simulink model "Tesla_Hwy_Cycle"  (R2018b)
settings: Solver=VariableStepAuto  StartTime=0.0  StopTime=765  FixedStep=1e-3  RelTol=1e-3
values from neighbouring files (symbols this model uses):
  B = 0    [Tesla_Initialization.m]    (also in PMSM_EV_init_v2.m; Leaf_Initialization.m)
  J = 0.3    [Tesla_Initialization.m]    (also in PMSM_EV_init_v2.m; Leaf_Initialization.m)
  P = 8    [Tesla_Initialization.m]    (also in PMSM_EV_init_v2.m; Iqbal Husain - Example12_1.m = V.*I; Leaf_Initialization.m)
  Rs = 0.046    [Tesla_Initialization.m]    (also in PMSM_EV_init_v2.m; Leaf_Initialization.m)
  Speed = [+0.000000E+00	+6.054730E+02	+1.210946E+03	+1.816419E+03	+2.421892E+03	+3.027365E+03	+3.632838E+03	+4.238311E+03	+5.775695E+03	+7.313079E+03	+8.850463E+03	+1.038785E+04	+1.192523E+04	+1.346262E+04	+1.500000E+04]    [PMSM_EV_init_v2.m]
  Tesla_id_axis = [-8.764242E+02	-7.790438E+02	-6.816633E+02	-5.842828E+02	-4.869024E+02	-3.895219E+02	-2.921414E+02	-1.947609E+02	-9.738047E+01	+0.000000E+00]    [Tesla_Initialization.m]
  Tesla_iq_axis = [+0.000000E+00	+9.738047E+01	+1.947609E+02	+2.921414E+02	+3.895219E+02	+4.869024E+02	+5.842828E+02	+6.816633E+02	+7.790438E+02	+8.764242E+02]    [Tesla_Initialization.m]
  Tesla_Ld = [+8.821895E-05	+8.924938E-05	+9.139742E-05	+9.462732E-05	+1.042993E-04	+1.207302E-04	+1.435858E-04	+1.651379E-04	+1.771179E-04	+1.815302E-04    [Tesla_Initialization.m]
  Tesla_Lq = [+2.750008E-04	+2.848007E-04	+2.919706E-04	+2.981362E-04	+3.048757E-04	+3.200995E-04	+3.552424E-04	+3.955550E-04	+4.296280E-04	+4.500669E-04    [Tesla_Initialization.m]
  Tesla_omega_axis = [+0.000000E+00	+6.292573E+01	+1.258515E+02	+1.887772E+02	+2.517029E+02	+3.146286E+02	+3.775544E+02	+4.404801E+02	+5.271540E+02	+6.138279E+02	+7.005019E+02	+7.871758E+02	+8.738497E+02	+9.605236E+02	+1.047198E+03]    [Tesla_Initialization.m]
  Tesla_phid = [-9.964313E-02	-8.749389E-02	-7.506085E-02	-6.231998E-02	-4.899731E-02	-3.359246E-02	-1.574417E-02	+5.955898E-03	+2.974036E-02	+5.474011E-02    [Tesla_Initialization.m]
  Tesla_phiq = [+1.577834E-05	+2.291095E-05	+1.626960E-05	+6.018524E-06	+7.523247E-06	+1.073346E-05	+2.148179E-05	+1.486713E-05	+9.491501E-06	-7.613491E-07    [Tesla_Initialization.m]
  Tesla_T = [+1.173389E-01	+1.514507E-01	+9.410508E-02	+2.983867E-02	+3.108232E-02	+3.547627E-02	+5.325126E-02	+2.456943E-02	+7.842834E-03	+0.000000E+00    [Tesla_Initialization.m]
  Tesla_torque_axis = [+0.000000E+00	+2.093141E+01	+4.186282E+01	+6.279422E+01	+8.372563E+01	+1.046570E+02	+1.255884E+02	+1.396842E+02	+1.571452E+02	+1.795502E+02	+2.098144E+02	+2.538064E+02	+3.242133E+02	+4.360097E+02]    [Tesla_Initialization.m]
  Torque = [+0.000000E+00	+7.333624E+00	+1.466725E+01	+2.200087E+01	+2.933450E+01	+3.666812E+01	+4.400174E+01	+5.043561E+01	+5.870849E+01	+6.980054E+01	+8.566293E+01	+1.107686E+02	+1.535327E+02	+2.089386E+02]    [PMSM_EV_init_v2.m]
undefined symbols (not defined in the file or in its folder): A1, B766, HEV_Param
libraries: fl_lib x18, nesl_utility x9, sdl_lib x4

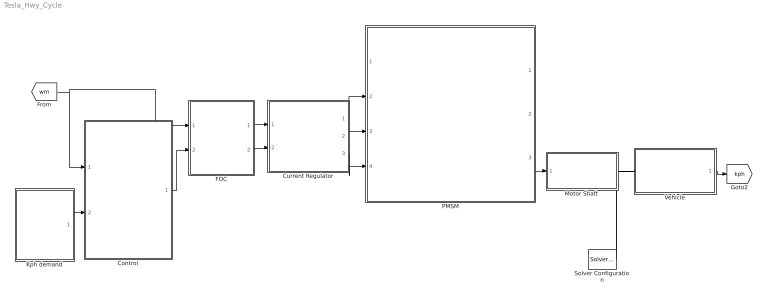
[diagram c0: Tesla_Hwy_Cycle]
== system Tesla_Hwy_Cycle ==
  Control : Subsystem
  Current Regulator : Subsystem
  FOC : Subsystem
  Kph demand : Subsystem
  Motor Shaft : Subsystem
  PMSM : Subsystem
  Solver Configuration : nesl_utility/Solver Configuration  PhysicalDomain=network_engine_domain  SubClassName=solver  LeftPortType=input  RightPortType=generic  Tones=[]  Harmonics=[]  SimulateNoise=off  Profile=off  UseLocalSampling=off  EnableSwitchedLinearOptims=on  FrequencyDomain=off  UseCCode=off  RelTol=0.001  AbsTol=1e-06  MinStep=1e-09  ToWorkspace=off  RevertToSquareIcSolve=off  NumHomotopyIterations=100  PhasorMode=off  PhasorModeNumHarmonics=1  DoDC=off  ResidualTolerance=1e-09  UseLocalSolver=off  LocalSolverChoice=NE_BACKWARD_EULER_ADVANCER  LocalSolverSampleTime=0.001  DoFixedCost=off  MaxNonlinIter=3  MaxModeIter=2  LinearAlgebra=auto  EquationFormulation=NE_TIME_EF  DelaysMemoryBudget=1024  AutomaticFiltering=on  FilteringTimeConstant=0.001  PartitionStorageMethod=AS_NEEDED  PartitionMemoryBudget=1024
  Vehicle : Subsystem
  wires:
  [wm] -> FOC/1(Speed), Control/1("rad/s ")
  FOC/2(Id_ref) -> Current Regulator/2(id_ref)
  PMSM/3(Torque (Nm)) -> Motor Shaft/1(In1)
  Current Regulator/2(Vb) -> PMSM/3(Vb)
  Control/1(Mot_TReq) -> FOC/2(Torque)
  Current Regulator/3(Vc) -> PMSM/4(Vc)
  Kph demand/1(Acc) -> Control/2(Acc)
  FOC/1(Iq_ref) -> Current Regulator/1(iq_ref)
  Vehicle/1(VehSpd) -> [kph]
  Current Regulator/1(Va) -> PMSM/2(Va)
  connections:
  Vehicle/LConn1 -- Solver Configuration/RConn1 -- Motor Shaft/RConn1

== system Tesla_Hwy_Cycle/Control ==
  "rad/s " : Inport
  Acc : Inport  Port=2
  Convert acceleration demand to motor speed demand. : Lookup  InputValues=[0 30]  Table=[0 10000]
  Gain : Gain  Gain=60/(2*pi)
  Motor Controller : Subsystem
  Mot_TReq : Outport
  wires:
  Motor Controller/1(M_Trq_Dem) -> Mot_TReq/1
  Convert acceleration demand to motor speed demand./1 -> Motor Controller/1(Mot_RPM_Dem)
  "rad/s "/1 -> Gain/1
  Acc/1 -> Convert acceleration demand to motor speed demand./1
  Gain/1 -> Motor Controller/2(Mot_RPM)

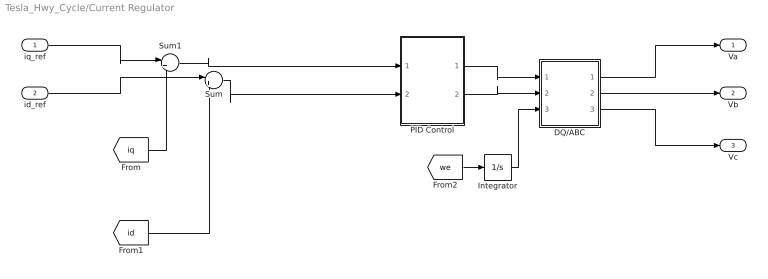
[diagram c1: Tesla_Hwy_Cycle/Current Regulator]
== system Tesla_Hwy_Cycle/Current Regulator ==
  iq_ref : Inport
  id_ref : Inport  Port=2
  DQ/ABC : Subsystem
  Integrator : Integrator
  PID Control : Subsystem
  Sum : Sum  Inputs=|+-
  Sum1 : Sum  Inputs=|+-
  Va : Outport
  Vb : Outport  Port=2
  Vc : Outport  Port=3
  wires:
  [iq] -> Sum1/2
  [id] -> Sum/2
  PID Control/1(Out1) -> DQ/ABC/1(Vq)
  Sum/1 -> PID Control/2(In3)
  PID Control/2(Out2) -> DQ/ABC/2(Vd)
  id_ref/1 -> Sum/1
  [we] -> Integrator/1
  iq_ref/1 -> Sum1/1
  Integrator/1 -> DQ/ABC/3(theta_rf)
  Sum1/1 -> PID Control/1(In1)
  DQ/ABC/1(Va) -> Va/1
  DQ/ABC/2("Vb ") -> Vb/1
  DQ/ABC/3("Vc ") -> Vc/1

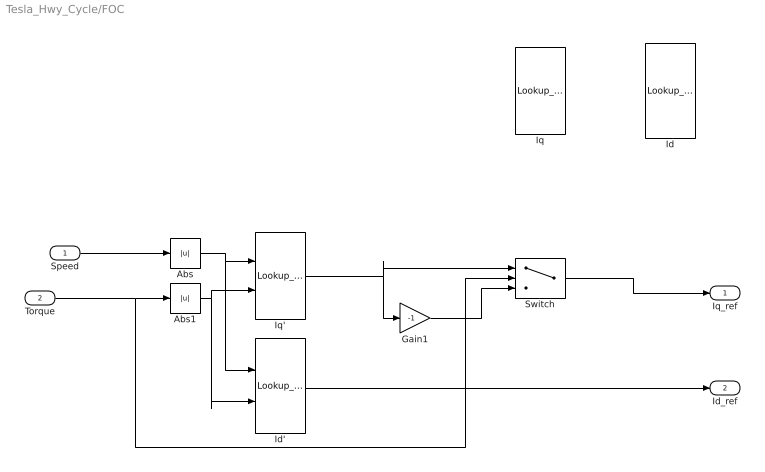
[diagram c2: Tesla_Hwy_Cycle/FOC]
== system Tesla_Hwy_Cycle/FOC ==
  Speed : Inport
  Torque : Inport  Port=2
  Abs : Abs
  Abs1 : Abs
  Gain1 : Gain  Gain=-1
  Id : Lookup_n-D  Commented=on  BreakpointsForDimension1=Speed  BreakpointsForDimension2=Torque  Table=Id_C'  InternalRulePriority=Speed  RndMeth=Simplest
  Id' : Lookup_n-D  BreakpointsForDimension1=Tesla_omega_axis  BreakpointsForDimension2=Tesla_torque_axis  Table=Tesla_Id'  InternalRulePriority=Speed  RndMeth=Simplest
  Iq : Lookup_n-D  Commented=on  BreakpointsForDimension1=Speed  BreakpointsForDimension2=Torque  Table=Iq_C'  InternalRulePriority=Speed  RndMeth=Simplest
  Iq' : Lookup_n-D  BreakpointsForDimension1=Tesla_omega_axis  BreakpointsForDimension2=Tesla_torque_axis  Table=Tesla_Iq'  InternalRulePriority=Speed  RndMeth=Simplest
  Switch : Switch  Criteria=u2 > Threshold
  Iq_ref : Outport
  Id_ref : Outport  Port=2
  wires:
  Abs/1 -> Id'/1, Iq'/1
  Abs1/1 -> Id'/2, Iq'/2
  Speed/1 -> Abs/1
  Switch/1 -> Iq_ref/1
  Torque/1 -> Switch/2, Abs1/1
  Gain1/1 -> Switch/3
  Iq'/1 -> Switch/1, Gain1/1
  Id'/1 -> Id_ref/1

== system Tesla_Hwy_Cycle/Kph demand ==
  From Spreadsheet3 : FromSpreadsheet  FileName=Highway_cycle.xlsx  Range=A1:B766  ExtrapolationBeforeFirstDataPoint=Hold first value
  Gain : Gain  Gain=1.6
  Vehicle Speed Controller : Subsystem
  Acc : Outport
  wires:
  From Spreadsheet3/1 -> Gain/1
  [kph] -> Vehicle Speed Controller/2(Veh Spd)
  Gain/1 -> Vehicle Speed Controller/1(Ref Spd)
  Vehicle Speed Controller/1(Acc) -> Acc/1

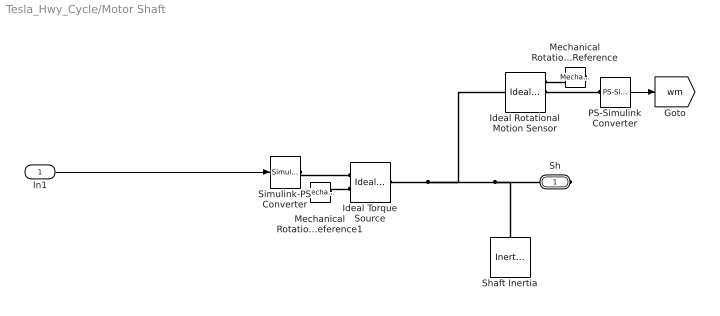
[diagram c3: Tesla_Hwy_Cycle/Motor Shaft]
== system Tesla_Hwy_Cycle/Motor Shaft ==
  In1 : Inport
  Ideal Rotational Motion Sensor : fl_lib/Mechanical/Mechanical Sensors/Ideal Rotational Motion Sensor  offset=0 rad
  Ideal Torque Source : fl_lib/Mechanical/Mechanical Sources/Ideal Torque Source
  Mechanical Rotational Reference : fl_lib/Mechanical/Rotational Elements/Mechanical Rotational Reference
  Mechanical Rotational Reference1 : fl_lib/Mechanical/Rotational Elements/Mechanical Rotational Reference
  PS-Simulink Converter : nesl_utility/PS-Simulink Converter  PhysicalDomain=network_engine_domain  SubClassName=ps_output  LeftPortType=input  RightPortType=output  PseudoPeriodic=off  Frequencies=[]  Unit=rad/s  AffineConversion=off
  Shaft Inertia : fl_lib/Mechanical/Rotational Elements/Inertia  inertia=HEV_Param.Motor.Shaft_Inertia kg*m^2  w_specify=on  w_priority=High  w=0 rad/s  w_nominal_specify=off  w_nominal_unit=rad/s  w_nominal_value=1  t_specify=off  t_priority=High  t=0 N*m  t_nominal_specify=off  t_nominal_unit=N*m  t_nominal_value=1
  Simulink-PS Converter : nesl_utility/Simulink-PS Converter  PhysicalDomain=network_engine_domain  SubClassName=ps_input  LeftPortType=input  RightPortType=output  PseudoPeriodic=off  Frequencies=[]  NoiseDistribution=none  NoiseParameters=[]  Unit=1  AffineConversion=off  FilteringAndDerivatives=zero  SimscapeFilterOrder=1  InputFilterTimeConstant=.001  UdotUserProvided=0
  Sh : PMIOPort  Side=Right
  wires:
  In1/1 -> Simulink-PS Converter/1
  PS-Simulink Converter/1 -> [wm]
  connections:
  Mechanical Rotational Reference1/LConn1 -- Ideal Torque Source/RConn2
  Ideal Torque Source/LConn1 -- Ideal Rotational Motion Sensor/LConn1 -- Shaft Inertia/LConn1 -- Sh/RConn1
  Simulink-PS Converter/RConn1 -- Ideal Torque Source/RConn1
  Mechanical Rotational Reference/LConn1 -- Ideal Rotational Motion Sensor/RConn1
  PS-Simulink Converter/LConn1 -- Ideal Rotational Motion Sensor/RConn2

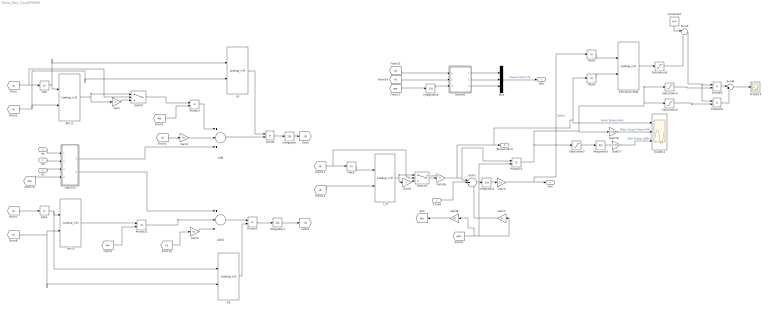
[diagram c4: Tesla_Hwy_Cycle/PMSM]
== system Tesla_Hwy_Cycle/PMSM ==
  T_load : Inport
  Va : Inport  Port=2
  Vb : Inport  Port=3
  Vc : Inport  Port=4
  ABC/DQ : Subsystem
  Abs{,1..2,5..6} (5 alike) : Abs
  Add : Sum  Inputs=+-+
  Add1 : Sum  Inputs=+--
  Constant2 : Constant  Value=1e-6
  DQ/ABC : Subsystem
  Divide : Product  Inputs=/*
  Divide1 : Product  Inputs=*/
  Divide4 : Product  Inputs=/*
  Efficiency Map : Lookup_n-D  BreakpointsForDimension1=Tesla_omega_axis  BreakpointsForDimension2=Tesla_torque_axis  Table=Tesla_eff'  ExtrapMethod=Clip  UseLastTableValue=on  InternalRulePriority=Speed  RndMeth=Simplest
  Gain : Gain  Gain=-1
  Gain1 : Gain  Gain=Rs
  Gain16 : Gain
  Gain17 : Gain  Gain=2.77778e-7
  Gain18 : Gain  Gain=1/1000
  Gain2 : Gain  Gain=Rs
  Gain3 : Gain  Gain=-1
  Gain4 : Gain  Gain=1/J
  Gain7 : Gain  Gain=B
  Gain8 : Gain  Gain=P/2
  Integrator{,1..2,4..5} (5 alike) : Integrator
  Ld : Lookup_n-D  BreakpointsForDimension1=Tesla_iq_axis  BreakpointsForDimension2=Tesla_id_axis  Table=Tesla_Ld  InternalRulePriority=Speed  RndMeth=Simplest
  Lq : Lookup_n-D  BreakpointsForDimension1=Tesla_iq_axis  BreakpointsForDimension2=Tesla_id_axis  Table=Tesla_Lq  InternalRulePriority=Speed  RndMeth=Simplest
  Mux : Mux  Inputs=3
  Product{,1,3,9} (4 alike) : Product
  Saturation2 : Saturate  UpperLimit=inf  LowerLimit=0
  Saturation3 : Saturate  UpperLimit=inf  LowerLimit=0
  Saturation4 : Saturate  UpperLimit=0  LowerLimit=-inf
  Saturation5 : Saturate  UpperLimit=inf  LowerLimit=0.1
  Scope12 : Scope  NumInputPorts=3
  Scope13 : Scope
  Sum1 : Sum  Inputs=|+--
  Sum5 : Sum  Inputs=|++
  Sum6 : Sum  Inputs=|++
  Switch : Switch  Criteria=u2 > Threshold
  Switch1 : Switch  Criteria=u2 > Threshold
  T_m : Lookup_n-D  BreakpointsForDimension1=Tesla_iq_axis  BreakpointsForDimension2=Tesla_id_axis  Table=Tesla_T  ExtrapMethod=Clip  UseLastTableValue=on  InternalRulePriority=Speed  RndMeth=Simplest
  phi_d : Lookup_n-D  BreakpointsForDimension1=Tesla_iq_axis  BreakpointsForDimension2=Tesla_id_axis  Table=Tesla_phid  InternalRulePriority=Speed  RndMeth=Simplest
  phi_q : Lookup_n-D  BreakpointsForDimension1=Tesla_iq_axis  BreakpointsForDimension2=Tesla_id_axis  Table=Tesla_phiq  InternalRulePriority=Speed  RndMeth=Simplest
  iabc : Outport
  wm : Outport  Port=2
  Torque (Nm) : Outport  Port=3
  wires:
  phi_d/1 -> Product1/1
  [iq] -> Abs1/1
  Divide1/1 -> Integrator1/1
  [we] -> ABC/DQ/4(omega_rf)
  T_m/1 -> Gain3/1, Switch1/1
  [id] -> Lq/2, phi_d/2
  [id] -> Ld/2, phi_q/2
  Vb/1 -> ABC/DQ/2(Vb)
  Integrator4/1 -> DQ/ABC/3(theta_rf)
  [id] -> Gain1/1
  Product1/1 -> Add1/2
  [we] -> Integrator4/1
  [iq] -> DQ/ABC/1(Iq)
  Abs/1 -> Ld/1, phi_q/1
  Vc/1 -> ABC/DQ/3(Vc)
  Gain4/1 -> Abs5/1, wm/1  "Speed"
  Divide/1 -> Integrator/1
  Add1/1 -> Divide1/1
  Gain1/1 -> Add/2
  [id] -> DQ/ABC/2(Id)
  Abs1/1 -> Lq/1, phi_d/1
  [iq] -> Gain2/1
  ABC/DQ/2("q ") -> Add1/1
  Integrator2/1 -> Gain4/1
  Ld/1 -> Divide/1
  [we] -> Product/2
  phi_q/1 -> Gain/1, Switch/1
  Product/1 -> Add/1
  Integrator1/1 -> [iq]
  ABC/DQ/1(d) -> Add/3
  T_load/1 -> Sum1/2
  [iq] -> Switch/2, Abs/1
  Add/1 -> Divide/2
  Switch1/1 -> Gain16/1  "Torque(Nm)"
  Switch/1 -> Product/1
  Sum1/1 -> Integrator2/1
  Abs2/1 -> T_m/1
  [we] -> Product1/2
  Va/1 -> ABC/DQ/1(Va)
  Integrator/1 -> [id]
  Gain/1 -> Switch/3
  Lq/1 -> Divide1/2
  Mux/1 -> iabc/1  "Phase Current (A)"
  Gain3/1 -> Switch1/3
  Gain2/1 -> Add1/3
  DQ/ABC/2("Ib ") -> Mux/2
  DQ/ABC/3("Ic ") -> Mux/3
  [wm] -> Gain7/1, Product3/2, Gain8/1
  Gain7/1 -> Sum1/3
  Gain8/1 -> [we]
  [id] -> T_m/2
  DQ/ABC/1(Ia) -> Mux/1
  [iq] -> Abs2/1, Switch1/2
  Gain16/1 -> Abs6/1, Scope12/1, Torque (Nm)/1, Product3/1, Sum1/1  "Motor Torque (Nm)"
  Integrator5/1 -> Gain17/1
  Gain18/1 -> Scope12/2  "Motor Output Power (kW)"
  Saturation2/1 -> Integrator5/1
  Gain17/1 -> Scope12/3  "Total Energy (kWhr)"
  Abs5/1 -> Efficiency Map/1
  Abs6/1 -> Efficiency Map/2
  Saturation4/1 -> Product9/2
  Saturation3/1 -> Divide4/2
  Product9/1 -> Sum6/2
  Sum6/1 -> Scope13/1
  Sum5/1 -> Product9/1, Divide4/1
  Constant2/1 -> Sum5/1
  Divide4/1 -> Sum6/1
  Product3/1 -> Saturation4/1, Saturation3/1, Gain18/1, Saturation2/1
  Efficiency Map/1 -> Saturation5/1
  Saturation5/1 -> Sum5/2

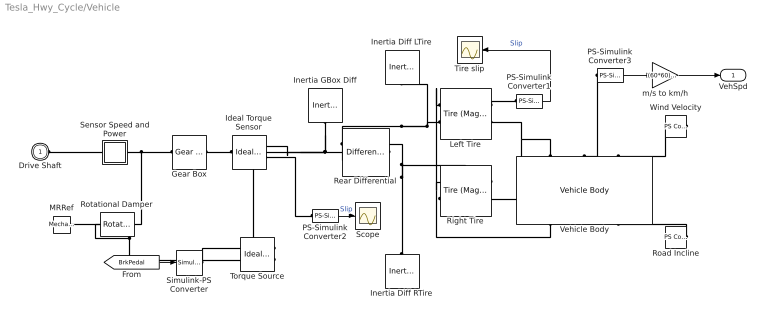
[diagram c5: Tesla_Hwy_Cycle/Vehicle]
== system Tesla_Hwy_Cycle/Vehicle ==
  Gear Box : fl_lib/Mechanical/Mechanisms/Gear Box  ratio=HEV_Param.Vehicle.Engine_Vehicle_Gear_Ratio  t_in_specify=off  t_in_priority=High  t_in=0 N*m  t_in_nominal_specify=off  t_in_nominal_unit=N*m  t_in_nominal_value=1  t_out_specify=off  t_out_priority=High  t_out=0 N*m  t_out_nominal_specify=off  t_out_nominal_unit=N*m  t_out_nominal_value=1
  Ideal Torque Sensor : fl_lib/Mechanical/Mechanical Sensors/Ideal Torque Sensor
  Inertia Diff LTire : fl_lib/Mechanical/Rotational Elements/Inertia  inertia=HEV_Param.Vehicle.Wheel_Inertia*2 kg*m^2  w_specify=on  w_priority=High  w=0 rad/s  w_nominal_specify=off  w_nominal_unit=rad/s  w_nominal_value=1  t_specify=off  t_priority=High  t=0 N*m  t_nominal_specify=off  t_nominal_unit=N*m  t_nominal_value=1
  Inertia Diff RTire : fl_lib/Mechanical/Rotational Elements/Inertia  inertia=HEV_Param.Vehicle.Wheel_Inertia*2 kg*m^2  w_specify=on  w_priority=High  w=0 rad/s  w_nominal_specify=off  w_nominal_unit=rad/s  w_nominal_value=1  t_specify=off  t_priority=High  t=0 N*m  t_nominal_specify=off  t_nominal_unit=N*m  t_nominal_value=1
  Inertia GBox Diff : fl_lib/Mechanical/Rotational Elements/Inertia  inertia=HEV_Param.Vehicle.Trans.Inertia kg*m^2  w_specify=on  w_priority=High  w=0 rad/s  w_nominal_specify=off  w_nominal_unit=rad/s  w_nominal_value=1  t_specify=off  t_priority=High  t=0 N*m  t_nominal_specify=off  t_nominal_unit=N*m  t_nominal_value=1
  Left Tire : sdl_lib/Tires & Vehicles/Tire (Magic Formula)  parameterization=1  F_z1=HEV_Param.Vehicle.Tire.Rated_Vertical_Load N  F_x1=HEV_Param.Vehicle.Tire.Rated_Peak_Long_Force N  kappa1=HEV_Param.Vehicle.Tire.Slip_At_Peak_Force  B_m=10  C_m=1.9  D_m=1  E_m=0.97  fz0=4e+3 N  p_Cx=1.685  p_Dx=[ 1.21 -0.037 ]  p_Ex=[ 0.344 0.095 -0.02 0 ]  p_Kx=[ 21.51 -0.163 0.245 ]  p_Hx=[ -0.002 0.002 ]  p_Vx=[ 0 0 ]  v_tr_thr=0.1 m/s  r_e=HEV_Param.Vehicle.Tire_Radius m  model_compliance=0  stiffness=1e+6 N/m  damping=1000 N/(m/s)  model_inertia=1  inertia=1e-2 kg*m^2  initial_velocity=0 rpm  model_resistance=1  resistance_model=1  coeff=0.015  p_tire=250e3 Pa  alpha=-0.003  beta=0.97  coeff_a=84e-4  coeff_b=6.2e-4 s/m  coeff_c=1.6e-4 s^2/m^2  v_thr=1e-3 m/s
  MRRef : fl_lib/Mechanical/Rotational Elements/Mechanical Rotational Reference
  PS-Simulink Converter1 : nesl_utility/PS-Simulink Converter  PhysicalDomain=network_engine_domain  SubClassName=ps_output  LeftPortType=input  RightPortType=output  PseudoPeriodic=off  Frequencies=[]  Unit=1  AffineConversion=off
  PS-Simulink Converter2 : nesl_utility/PS-Simulink Converter  PhysicalDomain=network_engine_domain  SubClassName=ps_output  LeftPortType=input  RightPortType=output  PseudoPeriodic=off  Frequencies=[]  Unit=1  AffineConversion=off
  PS-Simulink Converter3 : nesl_utility/PS-Simulink Converter  PhysicalDomain=network_engine_domain  SubClassName=ps_output  LeftPortType=input  RightPortType=output  PseudoPeriodic=off  Frequencies=[]  Unit=m/s  AffineConversion=off
  Rear Differential : sdl_lib/Gears/Differential  driveshaft_location=2  cd_ratio=1  friction_model=1  efficiency=[ 0.85 0.92 ]  mu_visc=[ 0 0 ] N*m/(rad/s)  pwr_thr=[ 0.001 0.001 ] W  carrier_inertia=0 kg*m^2  planet_inertia=0 kg*m^2  temperature_TLU=[ 280 300 320 ] K  efficiency_ss_TLU=[ 0.95 0.9 0.85 ]  efficiency_cd_TLU=[ 0.95 0.9 0.85 ]  thermal_mass=50 J/K  T_init=300 K
  Right Tire : sdl_lib/Tires & Vehicles/Tire (Magic Formula)  parameterization=1  F_z1=HEV_Param.Vehicle.Tire.Rated_Vertical_Load N  F_x1=HEV_Param.Vehicle.Tire.Rated_Peak_Long_Force N  kappa1=HEV_Param.Vehicle.Tire.Slip_At_Peak_Force  B_m=10  C_m=1.9  D_m=1  E_m=0.97  fz0=4e+3 N  p_Cx=1.685  p_Dx=[ 1.21 -0.037 ]  p_Ex=[ 0.344 0.095 -0.02 0 ]  p_Kx=[ 21.51 -0.163 0.245 ]  p_Hx=[ -0.002 0.002 ]  p_Vx=[ 0 0 ]  v_tr_thr=0.1 m/s  r_e=HEV_Param.Vehicle.Tire_Radius m  model_compliance=0  stiffness=1e+6 N/m  damping=1000 N/(m/s)  model_inertia=1  inertia=1e-2 kg*m^2  initial_velocity=0 rpm  model_resistance=1  resistance_model=1  coeff=0.015  p_tire=250e3 Pa  alpha=-0.003  beta=0.97  coeff_a=84e-4  coeff_b=6.2e-4 s/m  coeff_c=1.6e-4 s^2/m^2  v_thr=1e-3 m/s
  Road Incline : fl_lib/Physical Signals/Sources/PS Constant  constant=HEV_Param.Vehicle.Incline
  Rotational Damper : fl_lib/Mechanical/Rotational Elements/Rotational Damper  D=HEV_Param.Vehicle.Trans.Friction N*m/(rad/s)  w_specify=off  w_priority=High  w=0 rad/s  w_nominal_specify=off  w_nominal_unit=rad/s  w_nominal_value=1  t_specify=off  t_priority=High  t=0 N*m  t_nominal_specify=off  t_nominal_unit=N*m  t_nominal_value=1
  Scope : Scope
  Sensor Speed and Power : Subsystem
  Simulink-PS Converter : nesl_utility/Simulink-PS Converter  PhysicalDomain=network_engine_domain  SubClassName=ps_input  LeftPortType=input  RightPortType=output  PseudoPeriodic=off  Frequencies=[]  NoiseDistribution=none  NoiseParameters=[]  Unit=1  AffineConversion=off  FilteringAndDerivatives=zero  SimscapeFilterOrder=1  InputFilterTimeConstant=0.001  UdotUserProvided=1
  Tire slip : Scope
  Torque Source : fl_lib/Mechanical/Mechanical Sources/Ideal Torque Source
  Vehicle Body : sdl_lib/Tires & Vehicles/Vehicle Body  mass=HEV_Param.Vehicle.Mass kg  n_w=2  x_f=HEV_Param.Vehicle.Distance_CG_FrontAxle m  x_r=HEV_Param.Vehicle.Distance_CG_RearAxle m  y_c=HEV_Param.Vehicle.Distance_CG_Ground m  model_pitch=0  inertia=4000 kg*m^2  suspension_model=1  k_f=1e4 N/m  b_f=1e4 N/(m/s)  k_r=1e4 N/m  b_r=1e4 N/(m/s)  k_f_TLU=[-2000, -1000, 0, 1000, 2000] N  x_f_TLU=[-.4, -.2, 0, .2, .4] m  b_f_TLU=[-200, -100, 0, 100, 200] N  v_f_TLU=[-4, -2, 0, 2, 4] m/s  k_r_TLU=[-2000, -1000, 0, 1000, 2000] N  x_r_TLU=[-.4, -.2, 0, .2, .4] m  b_r_TLU=[-200, -100, 0, 100, 200] N  v_r_TLU=[-4, -2, 0, 2, 4] m/s  interp_method=simscape.enum.interpolation.linear  extrap_method=simscape.enum.extrapolation.linear  model_hardstop=0  upper_bound_f=.25 m  lower_bound_f=-.25 m  stop_k_f=1e6 N/m  stop_b_f=150 N/(m/s)  upper_bound_r=.25 m  lower_bound_r=-.25 m  stop_k_r=1e6 N/m  stop_b_r=150 N/(m/s)  initial_pitch=0 rad  initial_pitch_rate=0 rad/s  g=9.81 m/s^2  liftoff_warning=0  area=HEV_Param.Vehicle.Frontal_Area m^2  Cd=HEV_Param.Vehicle.Aero_Drag_Coeff  rho=1.18 kg/m^3  v_specify=on  v_priority=High  v=0 m/s  v_nominal_specify=off  v_nominal_unit=m/s  v_nominal_value=1
  Wind Velocity : fl_lib/Physical Signals/Sources/PS Constant  constant=0
  m/s to km/h : Gain  Gain=(60*60)/1000
  Drive Shaft : PMIOPort  Side=Left
  VehSpd : Outport
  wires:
  PS-Simulink Converter2/1 -> Scope/1  "Slip"
  PS-Simulink Converter3/1 -> m/s to km/h/1
  [BrkPedal] -> Simulink-PS Converter/1
  PS-Simulink Converter1/1 -> Tire slip/1  "Slip"
  m/s to km/h/1 -> VehSpd/1
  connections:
  Drive Shaft/RConn1 -- Sensor Speed and Power/LConn1
  Vehicle Body/LConn1 -- Right Tire/RConn2 -- Left Tire/RConn2
  Sensor Speed and Power/RConn1 -- Rotational Damper/LConn1 -- Gear Box/LConn1
  Torque Source/RConn2 -- Rotational Damper/RConn1 -- MRRef/LConn1
  Road Incline/RConn1 -- Vehicle Body/RConn3
  Inertia GBox Diff/LConn1 -- Rear Differential/LConn1 -- Torque Source/LConn1 -- Ideal Torque Sensor/RConn1
  Left Tire/RConn1 -- PS-Simulink Converter1/LConn1
  Wind Velocity/RConn1 -- Vehicle Body/LConn3
  Simulink-PS Converter/RConn1 -- Torque Source/RConn1
  PS-Simulink Converter2/LConn1 -- Ideal Torque Sensor/RConn2
  PS-Simulink Converter3/LConn1 -- Vehicle Body/LConn2
  Ideal Torque Sensor/LConn1 -- Gear Box/RConn1
  Vehicle Body/RConn1 -- Right Tire/LConn1 -- Left Tire/LConn1
  Left Tire/LConn2 -- Rear Differential/RConn2 -- Inertia Diff LTire/LConn1
  Rear Differential/RConn1 -- Right Tire/LConn2 -- Inertia Diff RTire/LConn1

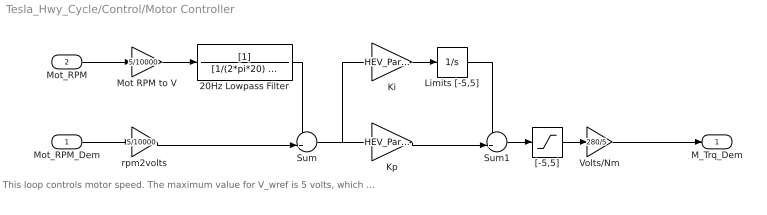
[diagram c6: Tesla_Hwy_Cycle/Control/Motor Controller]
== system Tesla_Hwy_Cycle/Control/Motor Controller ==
  note: This loop controls motor speed. The maximum value for V_wref is 5 volts, which is equivalent to a speed demand of 6500rpm.
  Mot_RPM_Dem : Inport
  Mot_RPM : Inport  Port=2
  20Hz Lowpass Filter : TransferFcn  Denominator=[1/(2*pi*20) 1]
  Ki : Gain  Gain=HEV_Param.Control.Mot.Ki
  Kp : Gain  Gain=HEV_Param.Control.Mot.Kp
  Limits [-5,5] : Integrator  LimitOutput=on  UpperSaturationLimit=5  LowerSaturationLimit=-5
  Mot RPM to V : Gain  Gain=5/10000
  Sum : Sum  Inputs=-+|
  Sum1 : Sum  Inputs=++|
  Volts/Nm : Gain  Gain=280/5
  "[-5,5]" : Saturate  UpperLimit=5  LowerLimit=-5
  rpm2volts : Gain  Gain=5/10000
  M_Trq_Dem : Outport
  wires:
  "[-5,5]"/1 -> Volts/Nm/1
  Mot_RPM/1 -> Mot RPM to V/1
  Sum1/1 -> "[-5,5]"/1
  Sum/1 -> Ki/1, Kp/1
  Ki/1 -> Limits [-5,5]/1
  Kp/1 -> Sum1/2
  Limits [-5,5]/1 -> Sum1/1
  20Hz Lowpass Filter/1 -> Sum/1
  rpm2volts/1 -> Sum/2
  Mot RPM to V/1 -> 20Hz Lowpass Filter/1
  Mot_RPM_Dem/1 -> rpm2volts/1
  Volts/Nm/1 -> M_Trq_Dem/1

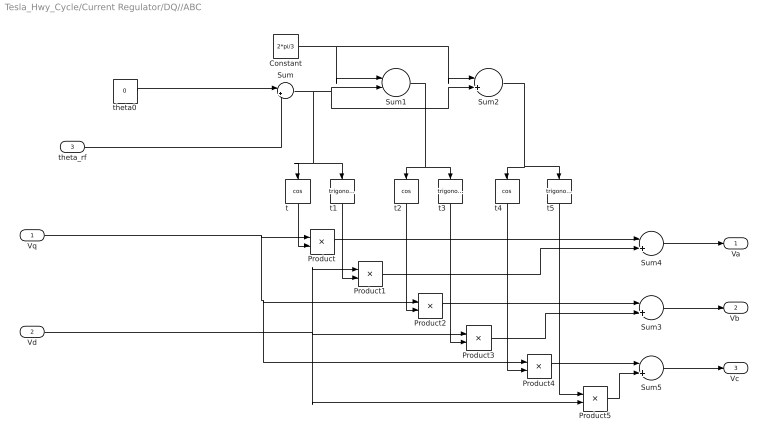
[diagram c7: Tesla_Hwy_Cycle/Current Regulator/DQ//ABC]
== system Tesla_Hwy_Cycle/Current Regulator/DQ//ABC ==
  Vq : Inport
  Vd : Inport  Port=2
  theta_rf : Inport  Port=3
  Constant : Constant  Value=2*pi/3
  Product{,1..5} (6 alike) : Product
  Sum{,2..5} (5 alike) : Sum  Inputs=|++
  Sum1 : Sum  Inputs=|-+
  t : Trigonometry  Operator=cos
  t1 : Trigonometry
  t2 : Trigonometry  Operator=cos
  t3 : Trigonometry
  t4 : Trigonometry  Operator=cos
  t5 : Trigonometry
  theta0 : Constant  Value=0
  Va : Outport
  "Vb " : Outport  Port=2
  "Vc " : Outport  Port=3
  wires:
  theta0/1 -> Sum/1
  Sum/1 -> t1/1, t/1, Sum2/2, Sum1/2
  Sum2/1 -> t5/1, t4/1
  Sum1/1 -> t2/1, t3/1
  t/1 -> Product/2
  Constant/1 -> Sum1/1, Sum2/1
  Product3/1 -> Sum3/2
  t1/1 -> Product1/2
  t3/1 -> Product3/2
  t2/1 -> Product2/2
  Sum4/1 -> Va/1
  Sum3/1 -> "Vb "/1
  theta_rf/1 -> Sum/2
  Vd/1 -> Product5/2, Product1/1, Product3/1
  Product/1 -> Sum4/1
  Product1/1 -> Sum4/2
  Product2/1 -> Sum3/1
  Vq/1 -> Product4/1, Product2/1, Product/1
  t4/1 -> Product4/2
  t5/1 -> Product5/1
  Product4/1 -> Sum5/1
  Product5/1 -> Sum5/2
  Sum5/1 -> "Vc "/1

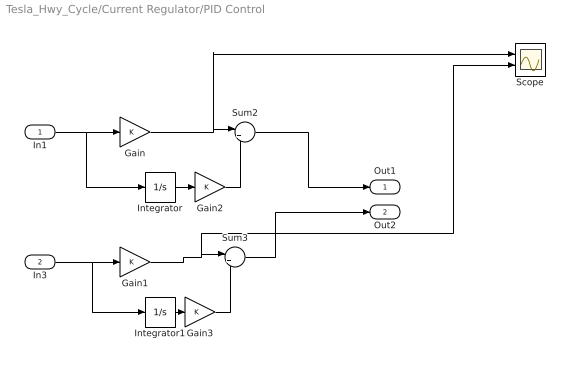
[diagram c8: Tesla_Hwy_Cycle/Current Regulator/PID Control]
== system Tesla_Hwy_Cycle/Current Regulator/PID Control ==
  In1 : Inport
  In3 : Inport  Port=2
  Gain{,1..3} (4 alike) : Gain
  Integrator : Integrator
  Integrator1 : Integrator
  Scope : Scope  NumInputPorts=2
  Sum2 : Sum  Inputs=|++
  Sum3 : Sum  Inputs=|++
  Out1 : Outport
  Out2 : Outport  Port=2
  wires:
  Integrator1/1 -> Gain3/1
  Gain1/1 -> Scope/2, Sum3/1
  Gain2/1 -> Sum2/2
  Gain/1 -> Scope/1, Sum2/1
  In1/1 -> Integrator/1, Gain/1
  Sum2/1 -> Out1/1
  In3/1 -> Integrator1/1, Gain1/1
  Integrator/1 -> Gain2/1
  Gain3/1 -> Sum3/2
  Sum3/1 -> Out2/1

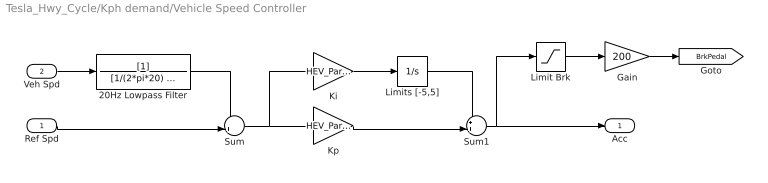
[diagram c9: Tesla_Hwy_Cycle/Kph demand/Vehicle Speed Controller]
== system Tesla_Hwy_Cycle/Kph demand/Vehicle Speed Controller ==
  Ref Spd : Inport
  Veh Spd : Inport  Port=2
  20Hz Lowpass Filter : TransferFcn  Denominator=[1/(2*pi*20) 1]
  Gain : Gain  Gain=200
  Ki : Gain  Gain=HEV_Param.Control.Veh_Spd.Ki
  Kp : Gain  Gain=HEV_Param.Control.Veh_Spd.Kp
  Limit Brk : Saturate  UpperLimit=0  LowerLimit=-inf
  Limits [-5,5] : Integrator  LimitOutput=on  UpperSaturationLimit=8  LowerSaturationLimit=-8
  Sum : Sum  Inputs=-+|
  Sum1 : Sum  Inputs=++|
  Acc : Outport
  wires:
  Ref Spd/1 -> Sum/2
  Veh Spd/1 -> 20Hz Lowpass Filter/1
  Sum/1 -> Ki/1, Kp/1
  Ki/1 -> Limits [-5,5]/1
  Kp/1 -> Sum1/2
  Limits [-5,5]/1 -> Sum1/1
  20Hz Lowpass Filter/1 -> Sum/1
  Limit Brk/1 -> Gain/1
  Gain/1 -> [BrkPedal]
  Sum1/1 -> Acc/1, Limit Brk/1

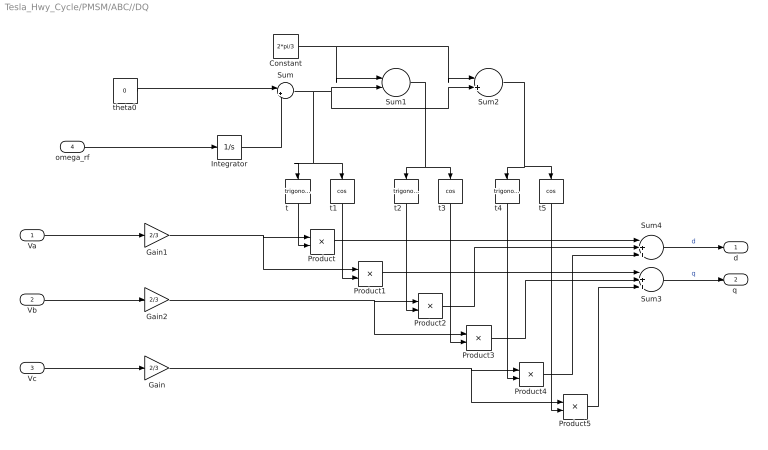
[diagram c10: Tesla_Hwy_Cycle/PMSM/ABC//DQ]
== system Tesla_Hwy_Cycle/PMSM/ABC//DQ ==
  Va : Inport
  Vb : Inport  Port=2
  Vc : Inport  Port=3
  omega_rf : Inport  Port=4
  Constant : Constant  Value=2*pi/3
  Gain : Gain  Gain=2/3
  Gain1 : Gain  Gain=2/3
  Gain2 : Gain  Gain=2/3
  Integrator : Integrator
  Product{,1..5} (6 alike) : Product
  Sum : Sum  Inputs=|++
  Sum1 : Sum  Inputs=|-+
  Sum2 : Sum  Inputs=|++
  Sum3 : Sum  Inputs=|+++
  Sum4 : Sum  Inputs=|+++
  t : Trigonometry
  t1 : Trigonometry  Operator=cos
  t2 : Trigonometry
  t3 : Trigonometry  Operator=cos
  t4 : Trigonometry
  t5 : Trigonometry  Operator=cos
  theta0 : Constant  Value=0
  d : Outport
  "q " : Outport  Port=2
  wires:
  theta0/1 -> Sum/1
  Sum/1 -> t1/1, t/1, Sum2/2, Sum1/2
  Sum2/1 -> t5/1, t4/1
  Integrator/1 -> Sum/2
  t4/1 -> Product4/2
  Sum1/1 -> t2/1, t3/1
  Product/1 -> Sum4/1
  t/1 -> Product/2
  Va/1 -> Gain1/1
  Constant/1 -> Sum1/1, Sum2/1
  Vc/1 -> Gain/1
  Product3/1 -> Sum3/2
  Gain2/1 -> Product3/1, Product2/1
  t5/1 -> Product5/2
  t1/1 -> Product1/2
  Gain/1 -> Product5/1, Product4/1
  Product1/1 -> Sum3/1
  Gain1/1 -> Product1/1, Product/1
  Product5/1 -> Sum3/3
  Product2/1 -> Sum4/2
  Product4/1 -> Sum4/3
  Vb/1 -> Gain2/1
  t3/1 -> Product3/2
  t2/1 -> Product2/2
  Sum4/1 -> d/1  "d"
  Sum3/1 -> "q "/1  "q"
  omega_rf/1 -> Integrator/1

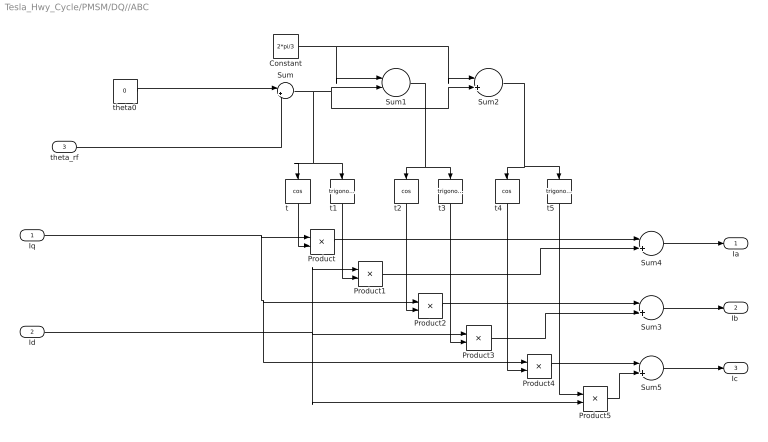
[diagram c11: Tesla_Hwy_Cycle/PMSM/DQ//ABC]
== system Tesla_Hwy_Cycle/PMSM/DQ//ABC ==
  Iq : Inport
  Id : Inport  Port=2
  theta_rf : Inport  Port=3
  Constant : Constant  Value=2*pi/3
  Product{,1..5} (6 alike) : Product
  Sum{,2..5} (5 alike) : Sum  Inputs=|++
  Sum1 : Sum  Inputs=|-+
  t : Trigonometry  Operator=cos
  t1 : Trigonometry
  t2 : Trigonometry  Operator=cos
  t3 : Trigonometry
  t4 : Trigonometry  Operator=cos
  t5 : Trigonometry
  theta0 : Constant  Value=0
  Ia : Outport
  "Ib " : Outport  Port=2
  "Ic " : Outport  Port=3
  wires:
  theta0/1 -> Sum/1
  Sum/1 -> t1/1, t/1, Sum2/2, Sum1/2
  Sum2/1 -> t5/1, t4/1
  Sum1/1 -> t2/1, t3/1
  t/1 -> Product/2
  Constant/1 -> Sum1/1, Sum2/1
  Product3/1 -> Sum3/2
  t1/1 -> Product1/2
  t3/1 -> Product3/2
  t2/1 -> Product2/2
  Sum4/1 -> Ia/1
  Sum3/1 -> "Ib "/1
  theta_rf/1 -> Sum/2
  Id/1 -> Product5/2, Product1/1, Product3/1
  Product/1 -> Sum4/1
  Product1/1 -> Sum4/2
  Product2/1 -> Sum3/1
  Iq/1 -> Product4/1, Product2/1, Product/1
  t4/1 -> Product4/2
  t5/1 -> Product5/1
  Product4/1 -> Sum5/1
  Product5/1 -> Sum5/2
  Sum5/1 -> "Ic "/1

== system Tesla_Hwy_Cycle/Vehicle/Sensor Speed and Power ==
  Ideal Rotational Motion Sensor : fl_lib/Mechanical/Mechanical Sensors/Ideal Rotational Motion Sensor  offset=0 rad
  Ideal Torque Sensor : fl_lib/Mechanical/Mechanical Sensors/Ideal Torque Sensor
  Mechanical Rotational Reference : fl_lib/Mechanical/Rotational Elements/Mechanical Rotational Reference
  PS-Simulink Converter : nesl_utility/PS-Simulink Converter  PhysicalDomain=network_engine_domain  SubClassName=ps_output  LeftPortType=input  RightPortType=output  PseudoPeriodic=off  Frequencies=[]  Unit=N*m  AffineConversion=off
  PS-Simulink Converter1 : nesl_utility/PS-Simulink Converter  PhysicalDomain=network_engine_domain  SubClassName=ps_output  LeftPortType=input  RightPortType=output  PseudoPeriodic=off  Frequencies=[]  Unit=rad/s  AffineConversion=off
  Product : Product
  W2kW : Gain  Gain=0.001
  B : PMIOPort  Side=Left
  F : PMIOPort  Port=2  Side=Right
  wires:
  W2kW/1 -> [Pm_vehicle]
  Product/1 -> W2kW/1
  PS-Simulink Converter/1 -> Product/1
  PS-Simulink Converter1/1 -> Product/2
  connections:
  Mechanical Rotational Reference/LConn1 -- Ideal Rotational Motion Sensor/RConn1
  Ideal Rotational Motion Sensor/LConn1 -- F/RConn1 -- Ideal Torque Sensor/RConn1
  B/RConn1 -- Ideal Torque Sensor/LConn1
  PS-Simulink Converter/LConn1 -- Ideal Torque Sensor/RConn2
  PS-Simulink Converter1/LConn1 -- Ideal Rotational Motion Sensor/RConn2
